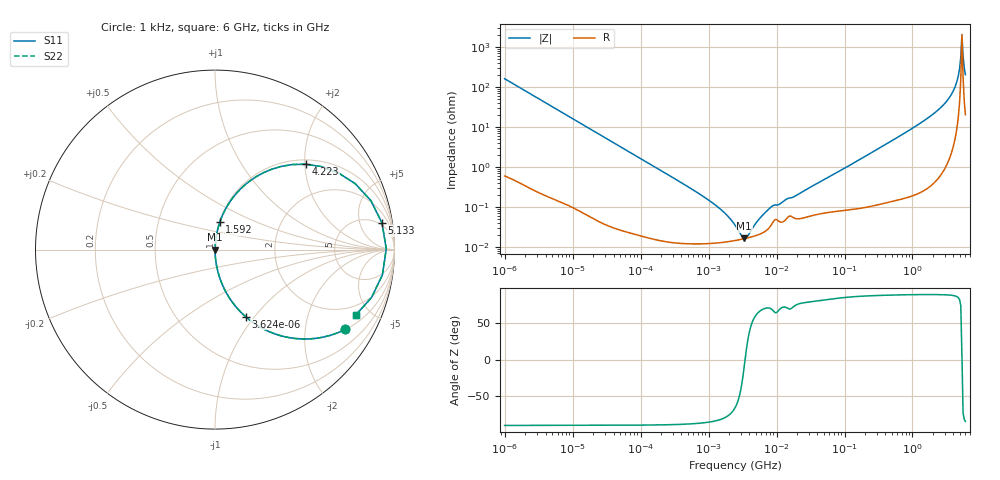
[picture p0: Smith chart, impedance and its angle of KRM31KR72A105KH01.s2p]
!Murata Part Number: KRM31KR72A105KH01
!These Parameters are Measured in Series Mode Connection
!Data Generated on Jan 08, 2026
!  o--ll--o
!Port1  Port2
!  o------o
!Operation Temp=25[degC], DC Bias Voltage=0[V]
!Freq. Start=1000[Hz] Stop=6[GHz] 401[Steps]
# Hz S RI R 50
!Freq.(Hz) S11(Real) S11(Imag) S21(Real) S21(Imag) S12(Real) S12(Imag) S22(Real) S22(Imag)
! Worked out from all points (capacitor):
!   401 points, 1 kHz to 6 GHz, reference 50 ohm
!   read as one part in series: C = 977 nF near 1.081 kHz
!   lowest |Z| = 16.6 mohm at 3.347 MHz (marker M1)
!   series resonance near 3.445 MHz, so ESL is about 2.2 nH
!   S11 on the Smith chart (normalised r, x): 1 kHz: 1.01, -3.26; 3.624 kHz: 1.00, -0.90; 1.592 GHz: 1.01, +0.32; 4.223 GHz: 1.10, +2.02; 5.133 GHz: 4, +11; 6 GHz: 1.41, -4.08
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1000  0.7253 -0.4445  0.2747 0.4445  0.2747 0.4445  0.7253 -0.4445
1867  0.4332 -0.4934  0.5668 0.4934  0.5668 0.4934  0.4332 -0.4934
3624  0.17 -0.3734  0.83 0.3734  0.83 0.3734  0.17 -0.3734
13657  0.015 -0.1183  0.985 0.1183  0.985 0.1183  0.015 -0.1183
186501  0.000227 -0.00885  0.9998 0.00885  0.9998 0.00885  0.000227 -0.00885
1122453  0.000127 -0.00131  0.9999 0.00131  0.9999 0.00131  0.000127 -0.00131
1792721  0.000136 -0.000664  0.9999 0.000664  0.9999 0.000664  0.000136 -0.000664
2449490  0.000148 -0.000327  0.9999 0.000327  0.9999 0.000327  0.000148 -0.000327
3346869  0.000164 -2.69e-05  0.9998 2.69e-05  0.9998 2.69e-05  0.000164 -2.69e-05
3762485  0.000172 8.25e-05  0.9998 -8.25e-05  0.9998 -8.25e-05  0.000172 8.25e-05
8210741  0.000345 0.000934  0.9997 -0.000934  0.9997 -0.000934  0.000345 0.000934
3.345153e7  0.000629 0.0033  0.9994 -0.0033  0.9994 -0.0033  0.000629 0.0033
4.568318e8  0.00312 0.042  0.9969 -0.042  0.9969 -0.042  0.00312 0.042
1.59224e9  0.0272 0.1541  0.9728 -0.1541  0.9728 -0.1541  0.0272 0.1541
3.090863e9  0.1562 0.351  0.8438 -0.351  0.8438 -0.351  0.1562 0.351
3.612945e9  0.2719 0.4293  0.7281 -0.4293  0.7281 -0.4293  0.2719 0.4293
4.223212e9  0.5064 0.4754  0.4936 -0.4754  0.4936 -0.4754  0.5064 0.4754
4.565976e9  0.6854 0.4288  0.3146 -0.4288  0.3146 -0.4288  0.6854 0.4288
5.132982e9  0.9305 0.1486  0.0695 -0.1486  0.0695 -0.1486  0.9305 0.1486
5.549585e9  0.9329 -0.1407  0.0671 0.1407  0.0671 0.1407  0.9329 -0.1407
5.770399e9  0.8718 -0.2674  0.1282 0.2674  0.1282 0.2674  0.8718 -0.2674
6e9  0.7851 -0.3636  0.2149 0.3636  0.2149 0.3636  0.7851 -0.3636
